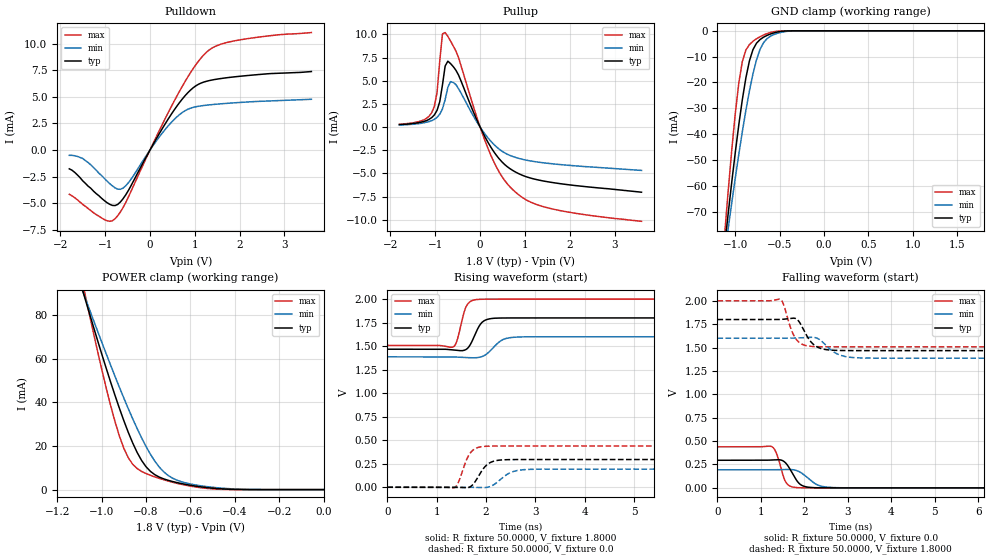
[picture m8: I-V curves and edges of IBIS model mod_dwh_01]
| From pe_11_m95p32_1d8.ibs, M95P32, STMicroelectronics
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|   Model mod_dwh_01
[Model]   mod_dwh_01
Model_type I/O
Polarity   Non-Inverting
Enable   Active-High
Vinl   =   0.540V
Vinh   =   1.260V
Vmeas  =   0.900V
Cref   =   30.0pF
C_comp   1.630pF   1.607pF   1.683pF
[Model Spec]
Vinl   0.540V  0.480V  0.600V  | <- for Vcc = 1.8V, 1.6V, 2.0V
Vinh   1.260V  1.120V  1.400V  | <- for Vcc = 1.8V, 1.6V, 2.0V
Vmeas  0.900V  0.800V  1.000V  | <- for Vcc = 1.8V, 1.6V, 2.0V
[Temperature Range]  25.0000   0.1050k   -40.0000
[Voltage Range]   1.8000V   1.6000V   2.0000V
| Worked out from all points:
|   slope of the pulldown table from 0 to 0.27 V, typ, clamps not added: 136 ohm
|   slope of the pullup table from 0 to 0.27 V, typ, clamps not added: 113 ohm
|   GND clamp passes 1 mA (typ) near -0.58 V on its own axis
|   POWER clamp passes 1 mA (typ) near -0.53 V on its own axis
|   rising waveform, R_fixture 50.0000, V_fixture 1.8000: 20-80 % time 187ps typ, 259ps min, 144ps max; typ from 1.47 V to 1.8 V
|   rising waveform, R_fixture 50.0000, V_fixture 0.0: 20-80 % time 234ps typ, 298ps min, 196ps max; typ from 0 V to 0.295 V
|   falling waveform, R_fixture 50.0000, V_fixture 0.0: 20-80 % time 236ps typ, 324ps min, 172ps max; typ from 0.295 V to 0 V
|   falling waveform, R_fixture 50.0000, V_fixture 1.8000: 20-80 % time 276ps typ, 347ps min, 223ps max; typ from 1.8 V to 1.47 V
[Pulldown]
|Voltage   I(typ)   I(min)   I(max)
-1.8V     -1.77mA    -500uA     -4.16mA
-1.5V     -2.9mA     -800uA     -5.12mA
-1.02V    -4.75mA    -2.66mA    -6.54mA
-840mV    -5.208mA   -3.37mA    -6.655mA
-660mV    -4.886mA   -3.696mA   -5.823mA
-540mV    -4.208mA   -3.356mA   -4.93mA
240mV     1.773mA    1.411mA    2.112mA
660mV     4.469mA    3.334mA    5.541mA
960mV     5.842mA    4.006mA    7.64mA
1.26V     6.464mA    4.216mA    9.195mA
1.92V     6.897mA    4.448mA    10.3mA
3.6V      7.38mA     4.77mA     11.05mA
[Pullup]
|Voltage   I(typ)   I(min)   I(max)
-1.8V     270uA      210uA      300uA
-1.08V    1.022mA    691uA      1.55mA
-960mV    1.813mA    1.051mA    3.765mA
-900mV    2.748mA    1.389mA    7.165mA
-840mV    4.548mA    1.964mA    10.06mA
-780mV    6.594mA    2.97mA     10.2mA
-660mV    6.854mA    4.91mA     9.291mA
-540mV    6.135mA    4.587mA    8.207mA
180mV     -1.687mA   -1.196mA   -2.362mA
720mV     -4.659mA   -3.16mA    -6.718mA
1.5V      -5.897mA   -3.906mA   -8.705mA
3.6V      -7.03mA    -4.68mA    -10.17mA
[GND_clamp]
|Voltage   I(typ)   I(min)   I(max)
-1.8V     -319.7mA   -274.4mA   -407.3mA
-1.12V    -83.64mA   -87.01mA   -79.32mA
-1.08V    -71.08mA   -76.85mA   -62.45mA
-1V       -47.38mA   -57.28mA   -32.33mA
-960mV    -36.55mA   -47.99mA   -20.38mA
-920mV    -26.73mA   -39.15mA   -11.92mA
-840mV    -11.67mA   -23.32mA   -5.34mA
-760mV    -4.801mA   -11.23mA   -3.081mA
-720mV    -3.384mA   -7.183mA   -2.279mA
-640mV    -1.748mA   -2.99mA    -1.048mA
-440mV    -85.93uA   -314uA     -8.035uA
1.8V      367pA      1.678uA    95.55pA
[POWER_clamp]
|Voltage   I(typ)   I(min)   I(max)
-1.8V     354.3mA    299.2mA    462.7mA
-1.08V    89.41mA    89.52mA    92.12mA
-1.06V    82.53mA    84.01mA    82.65mA
-980mV    55.86mA    62.44mA    46.9mA
-920mV    37.35mA    46.96mA    24.63mA
-880mV    26.31mA    37.17mA    14.66mA
-840mV    17.07mA    28.03mA    9.669mA
-800mV    10.51mA    19.82mA    7.37mA
-740mV    5.731mA    10.32mA    5.151mA
-640mV    2.77mA     3.598mA    2.408mA
-420mV    154.7uA    391.9uA    29.01uA
0V        367pA      12.25nA    169pA
[Ramp]
| variable   typ   min   max
dV/dt_r   0.1770/0.2926n   0.1156/0.4434n   0.2634/0.2414n
dV/dt_f   0.1994/0.4224n   0.1282/0.5939n   0.2952/0.3113n
R_load = 50.0000
[Rising Waveform]
R_fixture= 50.0000
V_fixture= 1.8000
V_fixture_min= 1.6000
V_fixture_max= 2.0000
|time   V(typ)   V(min)   V(max)
0s        1.468V     1.386V     1.508V
1.328ns   1.46V      1.386V     1.491V
1.408ns   1.455V     1.384V     1.555V
1.6ns     1.467V     1.379V     1.925V
1.808ns   1.661V     1.378V     1.996V
1.904ns   1.746V     1.387V     1.999V
2.016ns   1.783V     1.419V     2V
2.32ns    1.799V     1.564V     2V
2.592ns   1.8V       1.596V     2V
8ns       1.8V       1.6V       2V
[Rising Waveform]
R_fixture= 50.0000
V_fixture= 0.0
V_fixture_min= 0.0
V_fixture_max= 0.0
|time   V(typ)   V(min)   V(max)
0s        5.894nV    739nV      954.2pV
1.352ns   48.91uV    236.7uV    -5mV
1.432ns   -943.1uV   248.5uV    43.46mV
1.592ns   -5.481mV   17.62uV    277.8mV
1.672ns   3.071mV    -431.2uV   358.5mV
1.936ns   192.6mV    -4.139mV   433.1mV
2.184ns   281.3mV    37.23mV    438.4mV
2.488ns   294mV      154.8mV    438.9mV
2.792ns   294.9mV    188mV      438.9mV
8ns       295mV      192.6mV    438.9mV
[Falling Waveform]
R_fixture= 50.0000
V_fixture= 0.0
V_fixture_min= 0.0
V_fixture_max= 0.0
|time   V(typ)   V(min)   V(max)
0s        295mV      192.6mV    438.9mV
1.248ns   298.2mV    192.8mV    441.3mV
1.36ns    301mV      194mV      366.5mV
1.568ns   266.9mV    196.7mV    65.04mV
1.792ns   102mV      189.1mV    4.267mV
1.888ns   43.86mV    171.7mV    1.345mV
2.016ns   13.58mV    130.4mV    296.2uV
2.304ns   1.046mV    31.23mV    12.89uV
2.592ns   84.09uV    5.197mV    1.892uV
8ns       361.6nV    1.006uV    503.8nV
[Falling Waveform]
R_fixture= 50.0000
V_fixture= 1.8000
V_fixture_min= 1.6000
V_fixture_max= 2.0000
|time   V(typ)   V(min)   V(max)
0s        1.8V       1.6V       2V
1.464ns   1.801V     1.6V       2.01V
1.528ns   1.804V     1.6V       1.953V
1.784ns   1.813V     1.602V     1.608V
1.88ns    1.776V     1.604V     1.556V
2.104ns   1.59V      1.609V     1.516V
2.408ns   1.487V     1.564V     1.509V
2.744ns   1.47V      1.435V     1.508V
3.128ns   1.468V     1.393V     1.508V
8ns       1.468V     1.386V     1.508V
